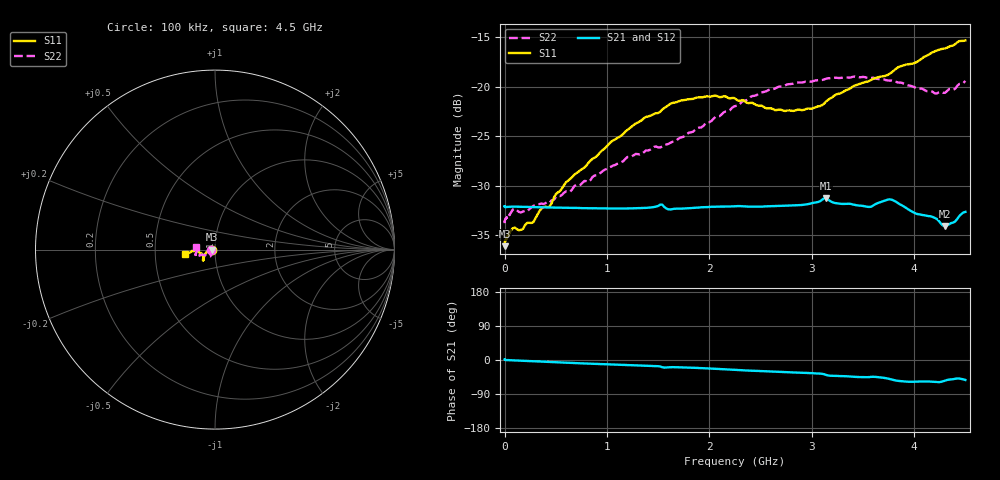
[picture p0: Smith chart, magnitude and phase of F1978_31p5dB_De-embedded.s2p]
! Integrated Device Technology
! Corporate Headquarters
! 6024 Silver Creek Valley Road
! San Jose, CA 95138  USA
! Phone:  1-408-284-8200
! Toll Free:  1-800-223-1366
! Webpage:  http://www.idt.com/
! Timing and RF Division
! 515 Groton Road, Suite 102
! Westford, MA 01886-6024
! Device:  F1978
! Description: 6-bit, 75 ohm, 0.5 dB Digital Step Attenuator
! Frequency:  5.0 MHz -  3.00 GHz
! Package:  4x4 mm QFN Plastic Package: 20 pin
! Ports:  2 RF, 11 DC
!  Pin  1  = D5 (16 dB)
!  Pin  2  = RF1  =  Port 1
!  Pin  3  = Serial Data In (DATA)
!  Pin  4  = Serial Clock (CLK)
!  Pin  5  = Serial Latch Enable (LE)
!  Pin  6  = VDD
!  Pin  7  = NC
!  Pin  8  = NC
!  Pin  9  = NC
!  Pin 10  = GND
!  Pin 11  = GND
!  Pin 12  = NC
!  Pin 13  = VMODE
!  Pin 14  = RF2  =  Port 2
!  Pin 15  = D4 (8 dB)
!  Pin 16  = D3 (4 dB)
!  Pin 17  = D2 (2 dB)
!  Pin 18  = NC
!  Pin 19  = D1 (1 dB)
!  Pin 20  = D0 (0.5 dB)
! State:  63
! Atten State:  31.5 dB
! Voltage:  +3.30 Volts
! Current:  0.561 mA
! Data:  The device was measured on a F1975 evaluation board which has
!  individual transmission lines to the RF pins.  Data was collected
!  using a calibrated network analyzer.  The evaluation board was
!  de-embedded using Automatic Fixture Removal (AFR).
!  The reference plane is the edge of the package pin.
! Misc:
!  Action Tracker AT0416
! Date Measured:  2018-02-08
! Date:  2018-03-26  MJV
! Note:
!  Integrated Device Technology supplies this data as a sample of measured
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# GHz S dB R 75
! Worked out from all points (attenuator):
!   291 points, 100 kHz to 4.5 GHz, reference 75 ohm
!   highest |S21| = -31.27 dB at 3.14 GHz (marker M1); lowest = -34.1 dB at 4.3 GHz (marker M2)
!   lowest |S11| = -36.1 dB at 100 kHz (marker M3), VSWR 1.03, Z = 72.7 - j0.0152 ohm
!   |S11| at or under -10 dB: start of sweep to end of sweep
!   |S22| runs from -33.8 to -19.0 dB; largest |S21 - S12| = 0.00019
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0.0001  -36.11 -179.6  -32.09 1.3  -32.08 1.2  -33.78 -179.2
0.005  -35.55 -178.3  -32.16 0.6  -32.17 0.3  -33.44 -177.6
0.08  -34.30 -176.4  -32.12 -0.9  -32.12 -0.9  -32.42 -169.5
0.16  -34.46 -177.2  -32.13 -2.1  -32.13 -2.1  -32.71 -160.1
0.28  -33.69 179.2  -32.16 -3.6  -32.16 -3.6  -32.04 -152.0
0.36  -32.31 179.6  -32.18 -4.5  -32.18 -4.5  -31.81 -144.4
0.44  -32.11 179.9  -32.20 -5.4  -32.20 -5.4  -31.72 -138.9
0.5  -30.86 -180.0  -32.22 -6.1  -32.21 -6.1  -31.17 -138.2
0.6  -29.65 -176.2  -32.24 -7.2  -32.24 -7.2  -30.58 -133.1
0.76  -28.30 -169.5  -32.27 -8.9  -32.27 -9.0  -29.71 -129.2
1.26  -23.87 -153.9  -32.28 -13.9  -32.28 -13.9  -26.94 -124.8
1.52  -22.54 -145.0  -31.92 -17.2  -31.91 -17.2  -26.14 -131.3
1.62  -21.72 -143.2  -32.40 -19.0  -32.40 -19.0  -25.67 -134.7
1.88  -21.10 -139.2  -32.22 -20.9  -32.22 -20.9  -24.20 -147.2
2.26  -21.29 -138.2  -32.07 -26.1  -32.07 -26.0  -21.96 -158.0
2.64  -22.37 -147.4  -32.05 -30.7  -32.05 -30.7  -20.20 -159.4
3.02  -22.15 -164.0  -31.73 -35.1  -31.72 -35.1  -19.43 -160.2
3.14  -21.49 -166.7  -31.27 -39.5  -31.26 -39.5  -19.20 -160.7
3.56  -19.43 -177.2  -32.15 -45.1  -32.15 -45.0  -19.16 -166.2
3.76  -18.71 -175.9  -31.38 -50.2  -31.38 -50.3  -19.40 -169.9
4.3  -16.15 -172.7  -34.07 -54.7  -34.05 -54.7  -20.63 177.0
4.5  -15.34 -172.3  -32.65 -52.7  -32.64 -52.7  -19.42 173.4
